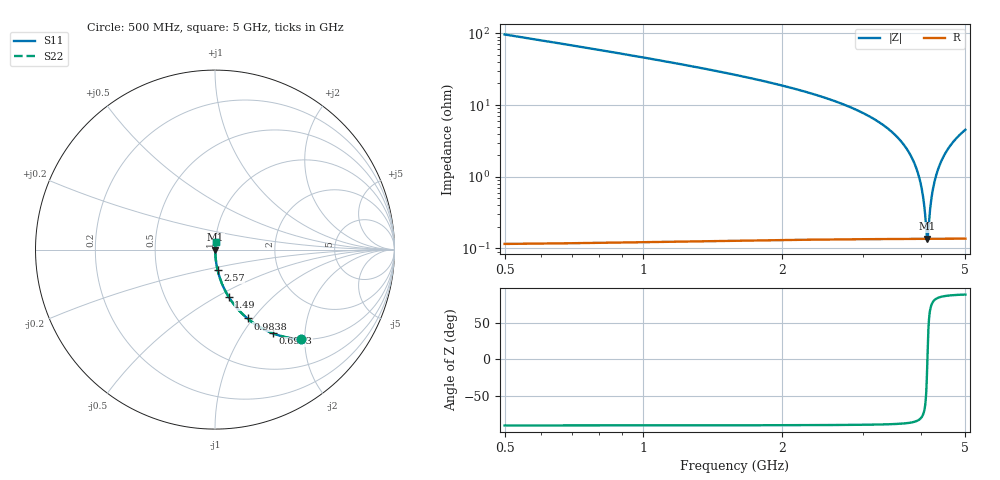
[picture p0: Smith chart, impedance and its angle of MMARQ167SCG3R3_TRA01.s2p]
! MMARQ167SCG3R3_TRA01  S-PARAMETER MODEL  ( General Type )
! Model Generated by TAIYO YUDEN Corporation (http://www.ty-top.com)
! Version 1.0
! TAIYO YUDEN Control No. 150305
! Copyright(c) 2015 TAIYO YUDEN CO.,LTD. All Rights Reserved.
! Product Description (link to TY-COMPAS)
! https://ds.yuden.co.jp/TYCOMPAS/or/detail?pn=MMARQ167SCG3R3BTRA01&u=M
! Products Name : Multilayer Ceramic Capacitors
! Characteristics :
!  Capacitance : 3.3 pF , Rated Voltage : 250V , TCC : CG / C0G
!  Case Size : 1.6 x 0.8 / 0.063 x 0.031 [mm/inch] , Thickness : 0.7 / 0.028 [mm/inch]
!  (Conditions: Temperature = 25 degC , DC Bias Current/Voltage = 0A / 0V)
! External Node Assignments :
!  1  o---| |---o  2
! GND o---------o GND
! Frequency Range : 500MHz  -  5GHz  [ 401 STEP ]
# MHz S RI R 50
! Freq[MHz].  S11 Real  S11 Imag  S21 Real  S21 Imag  S12 Real  S12 Imag  S22 Real  S22 Imag
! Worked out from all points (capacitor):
!   401 points, 500 MHz to 5 GHz, reference 50 ohm
!   read as one part in series: C = 3.25 pF near 522.5 MHz
!   lowest |Z| = 137 mohm at 4.134 GHz (marker M1)
!   series resonance near 4.135 GHz, so ESL is about 460 pH
!   S11 on the Smith chart (normalised r, x): 500 MHz: 1.00, -1.93; 691.2 MHz: 1.00, -1.38; 983.8 MHz: 1.00, -0.94; 1.49 GHz: 1.00, -0.57; 2.57 GHz: 1.00, -0.23; 5 GHz: 1.00, +0.09
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500  0.4819 -0.4991  0.5181 0.4991  0.5181 0.4991  0.4819 -0.4991
691.25  0.3216 -0.4662  0.6784 0.4662  0.6784 0.4662  0.3216 -0.4662
983.75  0.1811 -0.3838  0.8189 0.3838  0.8189 0.3838  0.1811 -0.3838
1253.75  0.1124 -0.3141  0.8876 0.3141  0.8876 0.3141  0.1124 -0.3141
1490  0.0765 -0.2635  0.9235 0.2635  0.9235 0.2635  0.0765 -0.2635
2007.5  0.0347 -0.1795  0.9653 0.1795  0.9653 0.1795  0.0347 -0.1795
2570  0.0147 -0.1149  0.9853 0.1149  0.9853 0.1149  0.0147 -0.1149
2750  0.011 -0.098  0.989 0.098  0.989 0.098  0.011 -0.098
3503.75  0.0029 -0.0392  0.9971 0.0392  0.9971 0.0392  0.0029 -0.0392
3762.5  0.00186 -0.0223  0.9981 0.0223  0.9981 0.0223  0.00186 -0.0223
3931.25  0.0015 -0.0119  0.9985 0.0119  0.9985 0.0119  0.0015 -0.0119
4032.5  0.0014 -0.00592  0.9986 0.00592  0.9986 0.00592  0.0014 -0.00592
4066.25  0.00138 -0.00395  0.9986 0.00395  0.9986 0.00395  0.00138 -0.00395
4111.25  0.00136 -0.00136  0.9986 0.00136  0.9986 0.00136  0.00136 -0.00136
4133.75  0.00136 -7.01e-05  0.9986 7.01e-05  0.9986 7.01e-05  0.00136 -7.01e-05
4156.25  0.00136 0.00121  0.9986 -0.00121  0.9986 -0.00121  0.00136 0.00121
4201.25  0.00138 0.00375  0.9986 -0.00375  0.9986 -0.00375  0.00138 0.00375
4257.5  0.00141 0.00689  0.9986 -0.00689  0.9986 -0.00689  0.00141 0.00689
4358.75  0.00152 0.0124  0.9985 -0.0124  0.9985 -0.0124  0.00152 0.0124
4516.25  0.0018 0.0208  0.9982 -0.0208  0.9982 -0.0208  0.0018 0.0208
4730  0.00238 0.0318  0.9976 -0.0318  0.9976 -0.0318  0.00238 0.0318
5000  0.0034 0.045  0.9966 -0.045  0.9966 -0.045  0.0034 0.045
